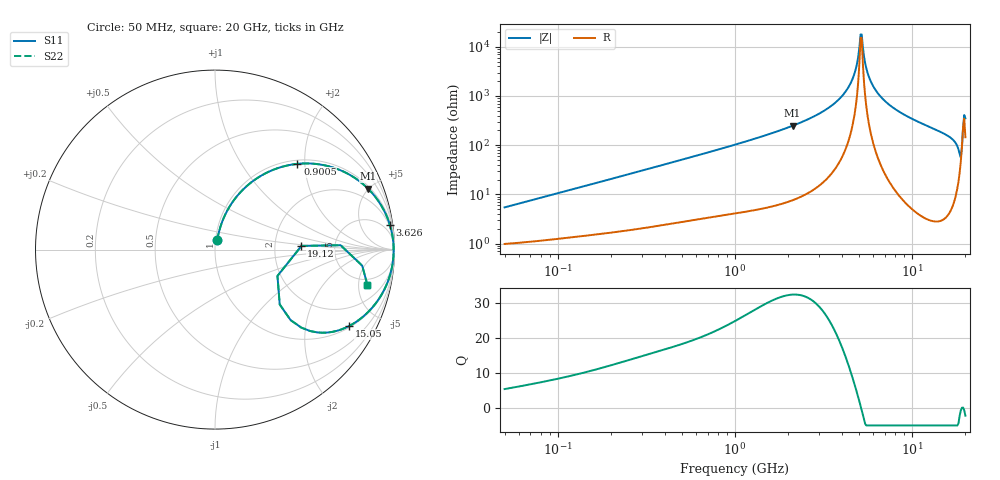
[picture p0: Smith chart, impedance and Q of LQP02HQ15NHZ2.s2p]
!Murata Part Number: LQP02HQ15NHZ2
!These Parameters are Measured in Series Mode Connection
!  o--[Z]--o
!Port1  Port2
!  o-------o
!Freq. Start=50[MHz] Stop=20[GHz], 401[Steps]
# Hz S RI R 50
!Freq.(Hz) S11(Real) S11(Imag) S21(Real) S21(Imag) S12(Real) S12(Imag) S22(Real) S22(Imag)
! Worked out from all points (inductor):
!   401 points, 50 MHz to 20 GHz, reference 50 ohm
!   read as one part in series: L = 17 nH near 51.52 MHz
!   highest Q = 32.5 at 2.115 GHz (marker M1), where L = 18.7 nH
!   self-resonance near 5.118 GHz
!   S11 on the Smith chart (normalised r, x): 50 MHz: 1.02, +0.11; 900.5 MHz: 1.08, +1.84; 3.626 GHz: 2, +14; 15.05 GHz: 1.06, -3.47; 19.12 GHz: 2.85, +0.15; 20 GHz: 3.90, -6.40
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5e7  0.0126 0.0525  0.9874 -0.0525  0.9874 -0.0525  0.0126 0.0525
1.364002e8  0.033 0.1356  0.967 -0.1356  0.967 -0.1356  0.033 0.1356
3.721004e8  0.1402 0.3179  0.8598 -0.3179  0.8598 -0.3179  0.1402 0.3179
9.00459e8  0.4595 0.4777  0.5405 -0.4777  0.5405 -0.4777  0.4595 0.4777
1e9  0.5123 0.4802  0.4877 -0.4802  0.4877 -0.4802  0.5123 0.4802
2.114743e9  0.8531 0.339  0.1469 -0.339  0.1469 -0.339  0.8531 0.339
2.728004e9  0.9248 0.248  0.0752 -0.248  0.0752 -0.248  0.9248 0.248
3.626126e9  0.974 0.1385  0.026 -0.1385  0.026 -0.1385  0.974 0.1385
4.149438e9  0.987 0.0857  0.013 -0.0857  0.013 -0.0857  0.987 0.0857
4.539627e9  0.9923 0.0503  0.00773 -0.0503  0.00773 -0.0503  0.9923 0.0503
4.81993e9  0.9943 0.0266  0.00567 -0.0266  0.00567 -0.0266  0.9943 0.0266
5.041459e9  0.9951 0.00887  0.00489 -0.00887  0.00489 -0.00887  0.9951 0.00887
5.194772e9  0.9953 -0.00299  0.00473 0.00299  0.00473 0.00299  0.9953 -0.00299
5.515528e9  0.9947 -0.0268  0.00528 0.0268  0.00528 0.0268  0.9947 -0.0268
5.856089e9  0.993 -0.0506  0.00701 0.0506  0.00701 0.0506  0.993 -0.0506
6.503449e9  0.9871 -0.0925  0.0129 0.0925  0.0129 0.0925  0.9871 -0.0925
7.442007e9  0.9738 -0.1467  0.0262 0.1467  0.0262 0.1467  0.9738 -0.1467
1.504638e10  0.7474 -0.4257  0.2526 0.4257  0.2526 0.4257  0.7474 -0.4257
1.774144e10  0.529 -0.4534  0.471 0.4534  0.471 0.4534  0.529 -0.4534
1.855685e10  0.3605 -0.3054  0.6395 0.3054  0.6395 0.3054  0.3605 -0.3054
1.912117e10  0.4819 0.0205  0.5181 -0.0205  0.5181 -0.0205  0.4819 0.0205
2e10  0.8491 -0.197  0.1509 0.197  0.1509 0.197  0.8491 -0.197
